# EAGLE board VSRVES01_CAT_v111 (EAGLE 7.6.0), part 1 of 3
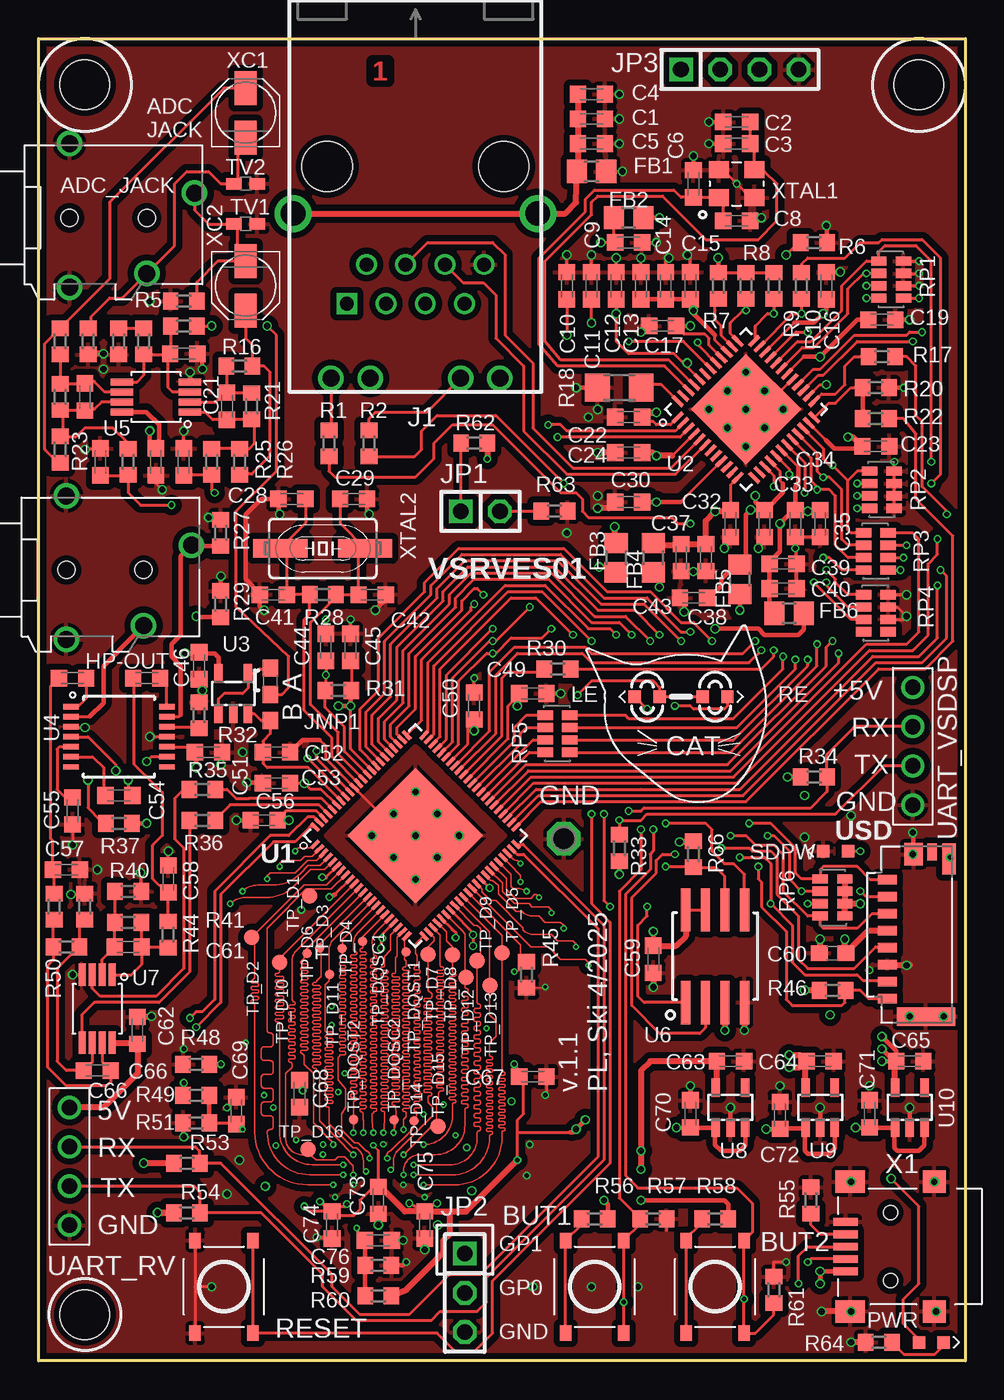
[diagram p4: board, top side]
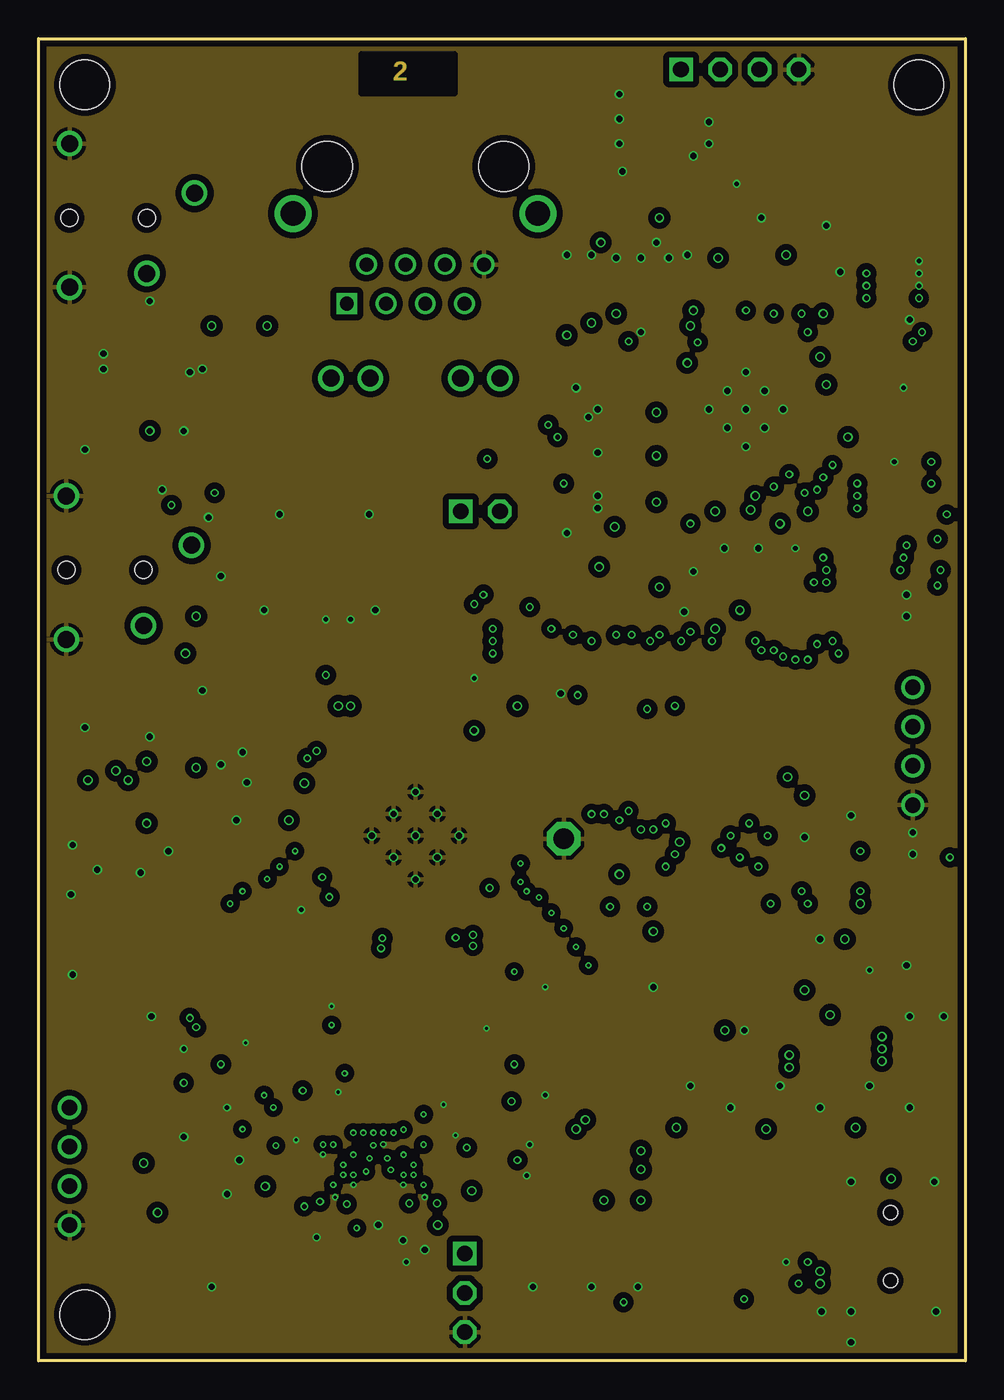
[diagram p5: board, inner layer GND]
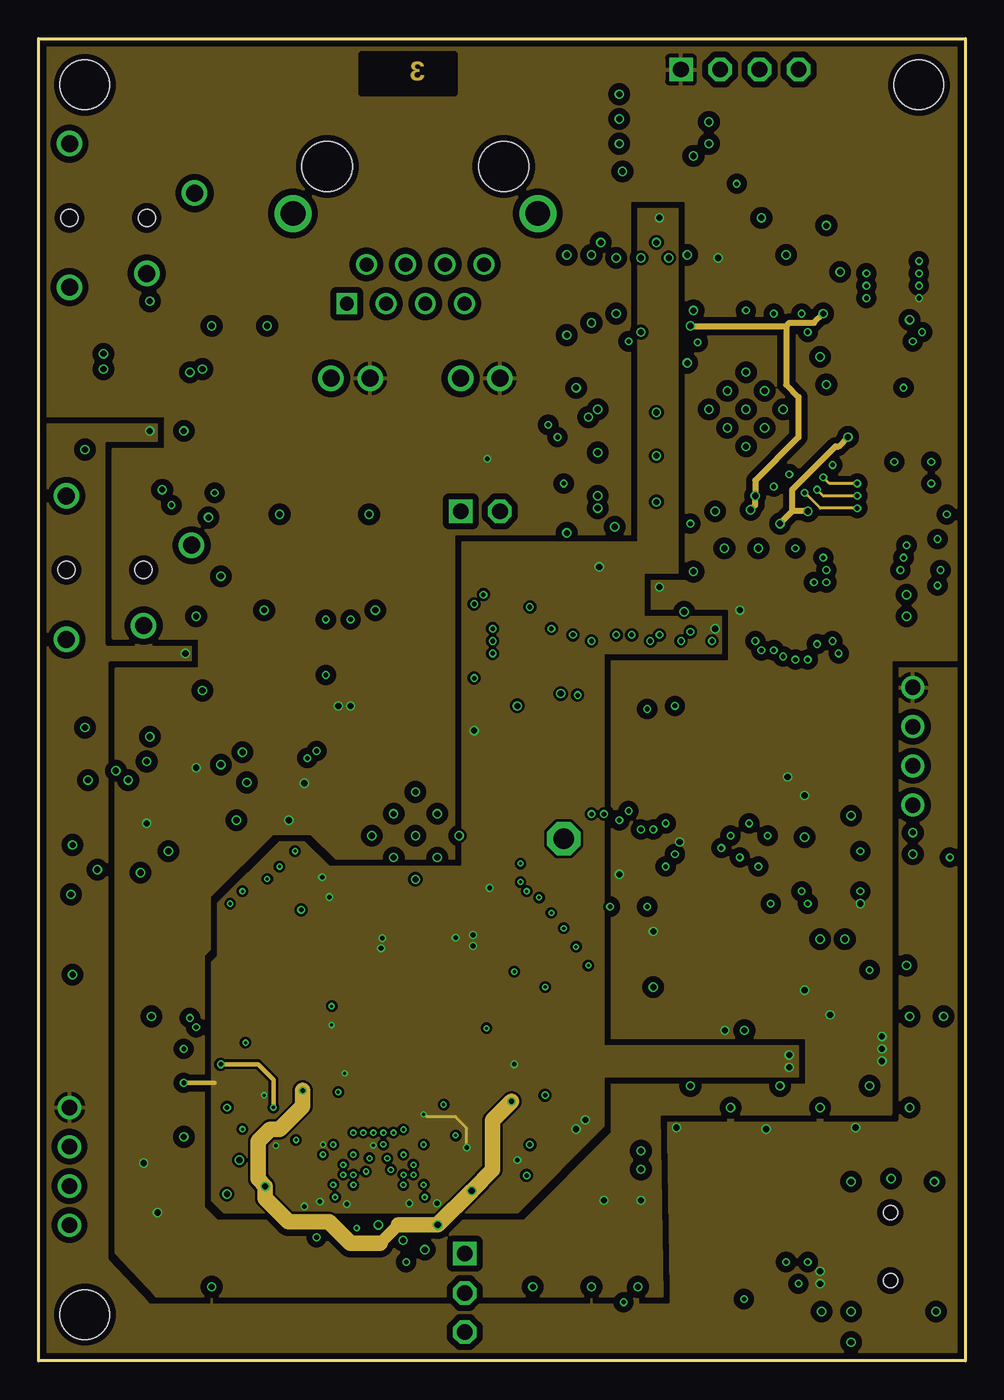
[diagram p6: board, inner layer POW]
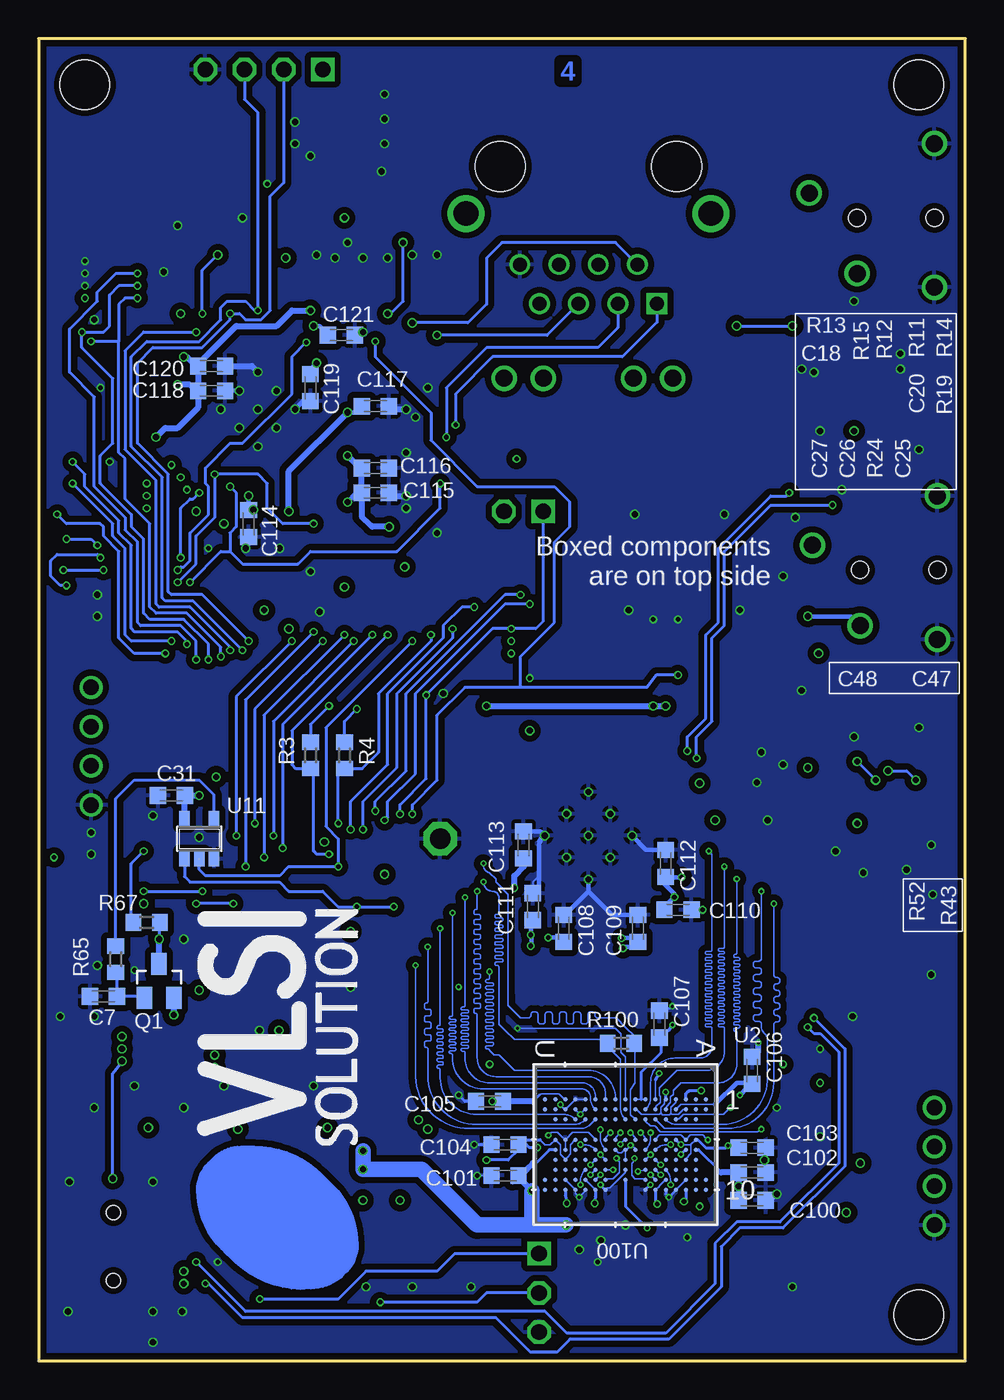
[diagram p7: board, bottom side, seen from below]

Size 60 x 85.6 mm. Coordinates in mm from the lower left corner, seen from the top.
Outline: 0,0 0,85.6 60,85.6 60,0 0,0
Copper layers (1*2+15*16): Top 0.035mm / dielectric 0.12mm / GND 0.0175mm / dielectric 1.2mm / POW 0.0175mm / dielectric 0.12mm / Bottom 0.035mm
Design rules "4L_JLC_tight_Eagle_Rule *": minimum track width 0.1mm, minimum drill 0.2mm, track to track 0.1mm, track to pad 0.1mm, pad to pad 0.15mm, via to via 0.2mm, smd to smd 0mil, copper to edge 6mil, drill to drill 12mil, minimum pad ring 0.1mm, minimum via ring 4mil, stop-mask expansion 2mil, vias tented up to drill 25mil, thermal gap 10mil
Holes 3.2 mm at 57,82.6 3,3 3,82.6
Milling: 4 lines

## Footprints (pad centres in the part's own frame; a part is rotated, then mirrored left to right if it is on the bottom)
SJ-43514B = drill 1.1: 1 8.1,1.6; 4 5,-3.6; 5 0,4.8; 6 0,-4.5 | hole 1.1: 0,0; 5,0
SW_SMD-SW-4_5.1X5.1X2.5_TS-1187A-C-E-B = smd 1 x 0.75: P1 -3,1.875; P2 3,1.875; S1 -3,-1.875; S2 3,-1.875
C0603K = smd 1.05 x 1.08: 1 -0.875,0; 2 0.875,0
C0603 = smd 1.1 x 1: 1 -0.85,0; 2 0.85,0
L0805 = smd 1.3 x 1.5: 1 -0.95,0; 2 0.95,0
JXD7 = drill 1.1: L1 -5.465,13.72; L2 -2.925,13.72; L3 2.925,13.72; L4 5.465,13.72 | drill 0.9 square: P1 4.445,8.89 | drill 0.9: P2 3.175,6.35; P3 1.905,8.89; P4 0.635,6.35; P5 -0.635,8.89; P6 -1.905,6.35; P7 -3.175,8.89; P8 -4.445,6.35 | drill 1.6: S1 7.925,3.05; S2 -7.925,3.05 | hole 3.25: 5.715,0; -5.715,0
0603X2 = smd 1.1 x 1: 1 -0.85,0; 2 0.85,0; 3 2.55,0
1X02 = drill 1.016 square: 1 -1.27,0 | drill 1.016 octagon: 2 1.27,0
1X03 = drill 1.016 square: 1 -2.54,0 | drill 1.016 octagon: 2 0,0; 3 2.54,0
1X04 = drill 1.016 square: 1 -3.81,0 | drill 1.016 octagon: 2 -1.27,0; 3 1.27,0; 4 3.81,0
LED_0603 = smd 0.8 x 0.8: A 0.8,0; C -0.8,0
SOT23 = smd 1.4 x 1: 1 1.1,-0.95; 2 1.1,0.95; 3 -1.1,0
R0603 = smd 1 x 1.1: 1 -0.85,0; 2 0.85,0
R1206 = smd 1.6 x 1.803: 1 -1.422,0; 2 1.422,0
RAS_ARR_1206 = smd 1 x 0.6: 1 -0.8,1.2; 2 0.8,1.2; 3 -0.8,0.4; 4 0.8,0.4; 5 -0.8,-0.4; 6 0.8,-0.4; 7 -0.8,-1.2; 8 0.8,-1.2
P1-13 = drill 1.321 pad 2.159 octagon: TP 0,0
TP10R = smd 1 x 1: TP 0,0
TP06R = smd 0.6 x 0.6: TP 0,0
0603 = smd 1.02 x 0.76: 1 -0.76,0; 2 0.76,0
QFN88_NEW2Q = smd 0.23 x 0.7: 1 -4.2,-5; 2 -3.8,-5; 3 -3.4,-5; 4 -3,-5; 5 -2.6,-5; 6 -2.2,-5; 7 -1.8,-5; 8 -1.4,-5; 9 -1,-5; 10 -0.6,-5; 11 -0.2,-5; 12 0.2,-5; 13 0.6,-5; 14 1,-5; 15 1.4,-5; 16 1.8,-5; 17 2.2,-5; 18 2.6,-5; 19 3,-5; 20 3.4,-5; 21 3.8,-5; 22 4.2,-5; 45 4.2,5; 46 3.8,5; 47 3.4,5; 48 3,5; 49 2.6,5; 50 2.2,5; 51 1.8,5; 52 1.4,5; 53 1,5; 54 0.6,5; 55 0.2,5; 56 -0.2,5; 57 -0.6,5; 58 -1,5; 59 -1.4,5; 60 -1.8,5; 61 -2.2,5; 62 -2.6,5; 63 -3,5; 64 -3.4,5; 65 -3.8,5; 66 -4.2,5 | smd 0.7 x 0.23: 23 5,-4.2; 24 5,-3.8; 25 5,-3.4; 26 5,-3; 27 5,-2.6; 28 5,-2.2; 29 5,-1.8; 30 5,-1.4; 31 5,-1; 32 5,-0.6; 33 5,-0.2; 34 5,0.2; 35 5,0.6; 36 5,1; 37 5,1.4; 38 5,1.8; 39 5,2.2; 40 5,2.6; 41 5,3; 42 5,3.4; 43 5,3.8; 44 5,4.2; 67 -5,4.2; 68 -5,3.8; 69 -5,3.4; 70 -5,3; 71 -5,2.6; 72 -5,2.2; 73 -5,1.8; 74 -5,1.4; 75 -5,1; 76 -5,0.6; 77 -5,0.2; 78 -5,-0.2; 79 -5,-0.6; 80 -5,-1; 81 -5,-1.4; 82 -5,-1.8; 83 -5,-2.2; 84 -5,-2.6; 85 -5,-3; 86 -5,-3.4; 87 -5,-3.8; 88 -5,-4.2 | smd 6.2 x 6.2: GNDPAD 0,0 | drill 0.4: P$1 -2,2; P$2 0,2; P$3 2,2; P$4 -2,0; P$5 0,0; P$6 2,0; P$7 -2,-2; P$8 0,-2; P$9 2,-2
48-VFQFN_7X7 = smd 0.9 x 0.25: 1 -3.5,2.75; 2 -3.5,2.25; 3 -3.5,1.75; 4 -3.5,1.25; 5 -3.5,0.75; 6 -3.5,0.25; 7 -3.5,-0.25; 8 -3.5,-0.75; 9 -3.5,-1.25; 10 -3.5,-1.75; 11 -3.5,-2.25; 12 -3.5,-2.75; 25 3.5,-2.75; 26 3.5,-2.25; 27 3.5,-1.75; 28 3.5,-1.25; 29 3.5,-0.75; 30 3.5,-0.25; 31 3.5,0.25; 32 3.5,0.75; 33 3.5,1.25; 34 3.5,1.75; 35 3.5,2.25; 36 3.5,2.75 | smd 0.25 x 0.9: 13 -2.75,-3.5; 14 -2.25,-3.5; 15 -1.75,-3.5; 16 -1.25,-3.5; 17 -0.75,-3.5; 18 -0.25,-3.5; 19 0.25,-3.5; 20 0.75,-3.5; 21 1.25,-3.5; 22 1.75,-3.5; 23 2.25,-3.5; 24 2.75,-3.5; 37 2.75,3.5; 38 2.25,3.5; 39 1.75,3.5; 40 1.25,3.5; 41 0.75,3.5; 42 0.25,3.5; 43 -0.25,3.5; 44 -0.75,3.5; 45 -1.25,3.5; 46 -1.75,3.5; 47 -2.25,3.5; 48 -2.75,3.5 | smd 5.05 x 5.05: 49 0,0 | drill 0.4: G1 -1.7,1.7; G2 0,1.7; G3 1.7,1.7; G4 -1.7,0; G5 0,0; G6 1.7,0; G7 -1.7,-1.7; G8 0,-1.7; G9 1.7,-1.7
SOT23-5 = smd 0.55 x 1.2: 1 -0.95,-1.3; 2 0,-1.3; 3 0.95,-1.3; 4 0.95,1.3; 5 -0.95,1.3
TSSOP-14_4.4MM = smd 0.35 x 1: 1 -1.95,-3.1; 2 -1.3,-3.1; 3 -0.65,-3.1; 4 0,-3.1; 5 0.65,-3.1; 6 1.3,-3.1; 7 1.95,-3.1; 8 1.95,3.1; 9 1.3,3.1; 10 0.65,3.1; 11 0,3.1; 12 -0.65,3.1; 13 -1.3,3.1; 14 -1.95,3.1
8-VSSOP = smd 0.45 x 1.45: 1 -0.975,-2.2; 2 -0.325,-2.2; 3 0.325,-2.2; 4 0.975,-2.2; 5 0.975,2.2; 6 0.325,2.2; 7 -0.325,2.2; 8 -0.975,2.2
SO-08M_WIDE = smd 0.6 x 2.8: 1 -1.905,-3; 2 -0.635,-3; 3 0.635,-3; 4 1.905,-3; 5 1.905,3; 6 0.635,3; 7 -0.635,3; 8 -1.905,3
SOT23-5L = smd 0.55 x 1.2: 1 -0.95,-1.3; 2 0,-1.3; 3 0.95,-1.3; 4 0.95,1.3; 5 -0.95,1.3
SOT23-5' = smd 0.69 x 0.99: 1 -0.95,-1.29; 2 0,-1.29; 3 0.95,-1.29; 4 0.95,1.3; 5 -0.95,1.3
FBGA134_ISI-L = smd 0.305 x 0.305: A1 -2.925,5.2; A2 -2.275,5.2; A9 2.275,5.2; A10 2.925,5.2; B1 -2.925,4.55; B2 -2.275,4.55; B3 -1.625,4.55; B5 -0.325,4.55; B6 0.325,4.55; B7 0.975,4.55; B8 1.625,4.55; B9 2.275,4.55; B10 2.925,4.55; C1 -2.925,3.9; C2 -2.275,3.9; C3 -1.625,3.9; C5 -0.325,3.9; C6 0.325,3.9; C7 0.975,3.9; C8 1.625,3.9; C9 2.275,3.9; C10 2.925,3.9; D1 -2.925,3.25; D2 -2.275,3.25; D3 -1.625,3.25; D5 -0.325,3.25; D6 0.325,3.25; D7 0.975,3.25; D8 1.625,3.25; D9 2.275,3.25; D10 2.925,3.25; E1 -2.925,2.6; E2 -2.275,2.6; E3 -1.625,2.6; E5 -0.325,2.6; E6 0.325,2.6; E7 0.975,2.6; E8 1.625,2.6; E9 2.275,2.6; E10 2.925,2.6; F1 -2.925,1.95; F2 -2.275,1.95; F3 -1.625,1.95; F5 -0.325,1.95; F6 0.325,1.95; F7 0.975,1.95; F8 1.625,1.95; F9 2.275,1.95; F10 2.925,1.95; G1 -2.925,1.3; G2 -2.275,1.3; G3 -1.625,1.3; G5 -0.325,1.3; G6 0.325,1.3; G7 0.975,1.3; G8 1.625,1.3; G9 2.275,1.3; G10 2.925,1.3; H1 -2.925,0.65; H2 -2.275,0.65; H3 -1.625,0.65; H5 -0.325,0.65; H6 0.325,0.65; J1 -2.925,0; J2 -2.275,0; J3 -1.625,0; J5 -0.325,0; J6 0.325,0; J7 0.975,0; J8 1.625,0; J9 2.275,0; K1 -2.925,-0.65; K2 -2.275,-0.65; K3 -1.625,-0.65; K5 -0.325,-0.65; K6 0.325,-0.65; L1 -2.925,-1.3; L2 -2.275,-1.3; L3 -1.625,-1.3; L5 -0.325,-1.3; L6 0.325,-1.3; L7 0.975,-1.3; L8 1.625,-1.3; L9 2.275,-1.3; L10 2.925,-1.3; M1 -2.925,-1.95; M2 -2.275,-1.95; M3 -1.625,-1.95; M5 -0.325,-1.95; M6 0.325,-1.95; M7 0.975,-1.95; M8 1.625,-1.95; M9 2.275,-1.95; M10 2.925,-1.95; N1 -2.925,-2.6; N2 -2.275,-2.6; N3 -1.625,-2.6; N5 -0.325,-2.6; N6 0.325,-2.6; N7 0.975,-2.6; N8 1.625,-2.6; N9 2.275,-2.6; N10 2.925,-2.6; P1 -2.925,-3.25; P2 -2.275,-3.25; P3 -1.625,-3.25; P5 -0.325,-3.25; P6 0.325,-3.25; P7 0.975,-3.25; P8 1.625,-3.25; P9 2.275,-3.25; P10 2.925,-3.25; R1 -2.925,-3.9; R2 -2.275,-3.9; R3 -1.625,-3.9; R5 -0.325,-3.9; R6 0.325,-3.9; R7 0.975,-3.9; R8 1.625,-3.9; R9 2.275,-3.9; R10 2.925,-3.9; T1 -2.925,-4.55; T2 -2.275,-4.55; T3 -1.625,-4.55; T5 -0.325,-4.55; T6 0.325,-4.55; T7 0.975,-4.55; T8 1.625,-4.55; T9 2.275,-4.55; T10 2.925,-4.55; U1 -2.925,-5.2; U2 -2.275,-5.2; U9 2.275,-5.2; U10 2.925,-5.2
4X1_2.54MM_CON = drill 1: P$1 0,0; P$2 2.54,0; P$3 5.08,0; P$4 7.62,0
47(309/571) = smd 0.6 x 1.25: 1 -3.55,-1.45; 2 -2.45,-1.45; 3 -1.35,-1.45; 4 -0.25,-1.45; 5 0.85,-1.45; 6 1.95,-1.45; 7 3.05,-1.45; 8 4.15,-1.45 | smd 1.2 x 3.79: 9 5.3,1.05 | smd 1.45 x 1.2: 10 -5.2,0.25 | smd 1.1 x 0.6: 11 -5.35,1.45 | smd 2 x 0.85: 12 -4.9,2.55
MINI_USB_KOREAN_HROPARTS_U-M-M5SS-W-2_C91144 = smd 1.6 x 0.5: 1 -4.15,-1.6; 2 -4.15,-0.8; 3 -4.15,0; 4 -4.15,0.8; 5 -4.15,1.6 | smd 1.9 x 1.45: G1 -3.85,-4.2; G2 -3.85,4.2 | smd 1.5 x 1.45: G3 1.6,-4.2; G4 1.6,4.2 | hole 0.9: -1.25,2.2; -1.25,-2.2
EC-SMD-44X44 = smd 2.2 x 1.4: + 1.6,0; - -1.6,0
3.2X2.5_CRYSTAL = smd 1.3 x 1.1: 1 -1.15,-0.9; 2 1.15,-0.9; 3 1.15,0.9; 4 -1.15,0.9
CSM-3X = smd 3.5 x 1.2: 1 -2.75,0; 2 2.75,0

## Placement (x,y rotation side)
$$U$1  [KISSA]  39.2,39.8 0 top
ADC_JACK  CON_3M5_4WAY_JACK-TH  [SJ-43514B]  2,74 0 top
BUT1  SW_SMD-C318887  [SW_SMD-SW-4_5.1X5.1X2.5_TS-1187A-C-E-B]  36,4.8 90 top
BUT2  SW_SMD-C318887  [SW_SMD-SW-4_5.1X5.1X2.5_TS-1187A-C-E-B]  43.8,4.8 90 top
C1  100nF  [C0603K]  35.8,80.4 0 top
C2  12p  [C0603K]  45.2,80.2 180 top
C3  12p  [C0603K]  45.2,78.8 180 top
C4  100nF  [C0603K]  35.8,82 0 top
C5  100nF  [C0603K]  35.8,78.8 0 top
C6  12p  [C0603K]  42.4,76.2 90 top
C7  100nF  [C0603K]  55.8,23.6 180 bottom
C8  12p  [C0603K]  45.2,73.8 0 top
C9  10u/6.3v  [C0603K]  38.2,72.4 0 top
C10  100nF  [C0603K]  34.2,69.6 90 top
C11  100nF  [C0603K]  35.8,69.6 90 top
C12  100nF  [C0603K]  37.4,69.6 90 top
C13  10u/6.3v  [C0603K]  39,69.6 90 top
C14  100nF  [C0603K]  40.6,69.6 90 top
C15  10nF  [C0603K]  42.2,69.6 90 top
C16  10nF  [C0603K]  51,69.6 90 top
C17  10nF  [C0603K]  40.4,67 180 top
C18  1uF  [C0603K]  9.4,65.2 0 top
C19  10nF  [C0603K]  54.6,67.4 0 top
C20  100pF  [C0603K]  3,62.4 270 top
C21  100pF  [C0603K]  12.2,61.8 270 top
C22  10nF  [C0603K]  38.2,61.1 180 top
C23  10nF  [C0603K]  54.2,59.2 0 top
C24  10nF  [C0603K]  38.2,58.8 180 top
C25  1n/NP0  [C0603K]  4,58.2 90 top
C26  100nF  [C0603K]  7.6,58.2 270 top
C27  1n/NP0  [C0603K]  9.4,58.2 90 top
C28  12p  [C0603K]  16.4,55.8 0 top
C29  12p  [C0603K]  20.4,55.8 180 top
C30  10nF  [C0603K]  38.2,55.6 180 top
C31  100nF  [C0603K]  51.4,36.6 180 bottom
C32  10nF  [C0603K]  44.8,54.2 270 top
C33  10nF  [C0603K]  47,54.2 270 top
C34  10nF  [C0603K]  49,54.2 270 top
C35  100nF  [C0603K]  50.6,54.2 270 top
C37  10u/6.3v  [C0603K]  41.6,52 270 top
C38  100nF  [C0603K]  43.2,52 270 top
C39  10u/6.3v  [C0603K]  48.2,51.6 0 top
C40  10u/6.3v  [C0603K]  48.2,50 0 top
C41  12p  [C0603K]  15.2,49.6 0 top
C42  12p  [C0603K]  21.6,49.6 180 top
C43  10u/6.3v  [C0603K]  42.4,49.4 180 top
C44  100nF  [C0603K]  18.6,46.2 90 top
C45  100nF  [C0603K]  20.2,46.2 90 top
C46  100nF  [C0603K]  10.4,45 270 top
C47  2.2uF  [C0603K]  2.2,44.2 0 top
C48  2.2uF  [C0603K]  7,44.2 0 top
C49  4.7uF  [C0603K]  32,43.2 0 top
C50  100nF  [C0603K]  28.2,42.4 90 top
C51  1uF  [C0603K]  11,39.4 0 top
C52  1uF  [C0603K]  15.4,39.4 0 top
C53  100nF  [C0603K]  15.4,37.4 180 top
C54  1uF  [C0603K]  5.2,36.6 180 top
C55  1uF  [C0603K]  2.2,35.6 270 top
C56  4.7uF  [C0603K]  14.6,35 180 top
C57  3.3n/NP0  [C0603K]  1.8,31.8 0 top
C58  3.3n/NP0  [C0603K]  8.4,31.2 90 top
C59  100nF  [C0603K]  39.8,26 270 top
C60  1uF  [C0603]  51.4,26.4 180 top
C61  1n/NP0  [C0603K]  5.8,26.8 0 top
C62  100nF  [C0603K]  6.4,21.4 90 top
C63  1uF  [C0603K]  44.8,19.4 0 top
C64  1uF  [C0603K]  50.6,19.4 0 top
C65  1uF  [C0603K]  56.4,19.4 0 top
C66  1n/NP0  [C0603K]  3.8,18.8 0 top
C67  100nF  [C0603K]  32,18.4 0 top
C68  100nF  [C0603K]  16.9,17.3 270 top
C69  100nF  [C0603K]  12.8,16.2 90 top
C70  1uF  [C0603K]  42.2,16 90 top
C71  1uF  [C0603K]  53.8,16 90 top
C72  1uF  [C0603K]  48,15.9 90 top
C73  100nF  [C0603K]  22,10.4 270 top
C74  100nF  [C0603K]  19,8.8 270 top
C75  10u/6.3v  [C0603K]  25,8.8 270 top
C76  100nF  [C0603K]  22,7.8 0 top
C100  10u/6.3v  [C0603K]  13.8,10.4 0 bottom
C101  100nF  [C0603K]  29.8,12 180 bottom
C102  100nF  [C0603K]  13.8,12.2 0 bottom
C103  100nF  [C0603K]  13.8,13.8 0 bottom
C104  100nF  [C0603K]  29.8,14 180 bottom
C105  100nF  [C0603K]  30.8,16.8 180 bottom
C106  100nF  [C0603K]  13.8,18.8 90 bottom
C107  100nF  [C0603K]  19.8,21.8 90 bottom
C108  100nF  [C0603K]  26,28 90 bottom
C109  100nF  [C0603K]  21.2,28 90 bottom
C110  4.7uF  [C0603K]  18.6,29.2 0 bottom
C111  100nF  [C0603K]  28,29.4 90 bottom
C112  4.7uF  [C0603K]  19.4,32.2 90 bottom
C113  100nF  [C0603K]  28.6,33.4 90 bottom
C114  100nF  [C0603K]  46.4,54.2 270 bottom
C115  100nF  [C0603K]  38.2,56.2 0 bottom
C116  10u/6.3v  [C0603K]  38.2,57.8 0 bottom
C117  10u/6.3v  [C0603K]  38.2,61.8 0 bottom
C118  10u/6.3v  [C0603K]  48.8,62.8 0 bottom
C119  10nF  [C0603K]  42.4,63 270 bottom
C120  10nF  [C0603K]  48.8,64.4 0 bottom
C121  10u/6.3v  [C0603K]  40.4,66.4 0 bottom
FB1  BLM21P221SG  [L0805]  35.8,77 0 top
FB2  BLM21P221SG  [L0805]  38.2,74 180 top
FB3  BLM21P221SG  [L0805]  37.4,52 90 top
FB4  BLM21P221SG  [L0805]  39.8,52 90 top
FB5  BLM21P221SG  [L0805]  45.4,50.6 90 top
FB6  BLM21P221SG  [L0805]  48.6,48.4 180 top
HP-OUT  CON_3M5_4WAY_JACK-TH  [SJ-43514B]  1.8,51.2 0 top
J1  JXD7-0V0XNL08NL  [JXD7]  24.4,77.33 180 top
JMP1  0R-JMPR  [0603X2]  15,44 270 top
JP1  dnc  [1X02]  28.6,55 0 top
JP2  3PIN  [1X03]  27.6,4.4 270 top
JP3  dnc  [1X04]  45.4,83.6 0 top
LE  amber  [LED_0603]  39.4,43 0 top
PWR  green  [LED_0603]  57.8,1.2 180 top
Q1  CJ3401A  [SOT23]  52.2,24.6 270 bottom
R1  1k  [R0603]  18.8,59.4 270 top
R2  1k  [R0603]  21.4,59.4 270 top
R3  1k  [R0603]  42.4,39.2 90 bottom
R4  1k  [R0603]  40.2,39.2 90 bottom
R5  100k  [R0603]  9.4,68.6 0 top
R6  1k  [R0603]  50.2,72.4 180 top
R7  10k  [R0603]  44,69.6 90 top
R8  10k  [R0603]  45.8,69.6 90 top
R9  10k  [R0603]  47.6,69.6 90 top
R10  10  [R0603]  49.4,69.6 90 top
R11  100k  [R0603]  3.2,66 90 top
R12  470k  [R0603]  5.2,66 90 top
R13  8k2  [R0603]  9.4,67 180 top
R14  8.2k  [R0603]  1.4,66 270 top
R15  470k  [R0603]  6.8,66 270 top
R16  8.2k  [R0603]  13,64.4 180 top
R17  10  [R0603]  54.6,65 0 top
R18  6.04k  [R1206]  37.6,63 180 top
R19  8.2k  [R0603]  1.4,62.4 270 top
R20  dnc  [R0603]  54.2,63 180 top
R21  8.2k  [R0603]  13.8,61.8 270 top
R22  10  [R0603]  54.2,61 0 top
R23  dnc  [R0603]  1.4,59 90 top
R24  100  [R0603]  5.8,58.2 270 top
R25  100  [R0603]  11.2,58.2 270 top
R26  dnc  [R0603]  13,58.2 90 top
R27  100k  [R0603]  11.8,53.6 270 top
R28  470k  [R0603]  18.4,49.6 0 top
R29  100k  [R0603]  11.8,49 270 top
R30  10  [R0603]  33.6,44.8 180 top
R31  100k  [R0603]  19.4,43.4 0 top
R32  82k  [R0603]  10.4,41.8 90 top
R33  10k  [R0603]  37.6,33.2 270 top
R34  10k  [R0603]  50.2,37.8 180 top
R35  1k  [R0603]  10.6,37 180 top
R36  1k  [R0603]  10.6,35 180 top
R37  10k  [R0603]  5.2,34.8 0 top
R40  470k  [R0603]  5.8,30.4 180 top
R41  1k  [R0603]  5.8,28.4 0 top
R43  1k  [R0603]  1,29.4 90 top
R44  1k  [R0603]  8.4,27.6 90 top
R45  10k  [R0603]  31.6,25 90 top
R46  10k  [R0603]  51.4,24 180 top
R48  240  [R0603]  10.2,19.2 0 top
R49  2k  [R0603]  10.2,17.2 180 top
R50  1k  [R0603]  1.8,26.8 180 top
R51  2k  [R0603]  10.2,15.4 0 top
R52  470k  [R0603]  3,29.4 270 top
R53  10k  [R0603]  9.6,12.8 180 top
R54  10k  [R0603]  9.6,9.6 180 top
R55  100k  [R0603]  50,10.4 90 top
R56  10k  [R0603]  36,9.2 0 top
R57  100k  [R0603]  39.8,9.2 180 top
R58  10k  [R0603]  43.8,9.2 0 top
R59  2k  [R0603]  22,6.2 180 top
R60  2k  [R0603]  22,4.2 0 top
R61  100k  [R0603]  47.6,4.6 270 top
R62  100k  [R0603]  28.2,59.4 0 top
R63  10k  [R0603]  33.4,55 180 top
R64  2k  [R0603]  54.4,1.2 0 top
R65  1k  [R0603]  55,26 270 bottom
R66  100k  [R0603]  42.4,32.8 90 top
R67  2k  [R0603]  53,28.4 180 bottom
R100  100  [R0603]  22.29,20.55 0 bottom
RE  green  [LED_0603]  43.8,43 180 top
RESET  SW_SMD-C318887  [SW_SMD-SW-4_5.1X5.1X2.5_TS-1187A-C-E-B]  12,4.8 90 top
RP1  10k  [RAS_ARR_1206]  55.2,70 180 top
RP2  1k  [RAS_ARR_1206]  54.6,56.4 180 top
RP3  10  [RAS_ARR_1206]  54.2,52.4 180 top
RP4  1k  [RAS_ARR_1206]  54.2,48.4 180 top
RP5  10  [RAS_ARR_1206]  33.6,40.6 180 top
RP6  10k  [RAS_ARR_1206]  51.4,30 0 top
SDPW  green  [LED_0603]  51.6,33 0 top
TP1  TPPAD1-13  [P1-13]  34,33.8 180 top
TP_D1  TPTP10R  [TP10R]  17.53,30.09 0 top
TP_D2  TPTP10R  [TP10R]  13.8,27.4 0 top
TP_D3  TPTP06R  [TP06R]  18.18,26.75 0 top
TP_D4  TPTP06R  [TP06R]  19.64,26.71 0 top
TP_D5  TPTP10R  [TP10R]  30,26.4 0 top
TP_D6  TPTP06R  [TP06R]  17.38,26.37 0 top
TP_D7  TPTP10R  [TP10R]  25.2,26.3 0 top
TP_D8  TPTP10R  [TP10R]  26.8,26.28 0 top
TP_D9  TPTP10R  [TP10R]  28.39,25.91 0 top
TP_D10  TPTP10R  [TP10R]  15.6,25.79 0 top
TP_D11  TPTP06R  [TP06R]  18.83,25.01 0 top
TP_D12  TPTP10R  [TP10R]  27.67,24.81 0 top
TP_D13  TPTP10R  [TP10R]  29.24,24.3 0 top
TP_D14  TPTP06R  [TP06R]  24.31,15.55 0 top
TP_D15  TPTP10R  [TP10R]  25.85,15.19 0 top
TP_D16  TPTP10R  [TP10R]  17.45,13.71 0 top
TP_DQSC1  TPTP06R  [TP06R]  20.99,27.16 0 top
TP_DQSC2  TPTP06R  [TP06R]  23,15.6 0 top
TP_DQST1  TPTP06R  [TP06R]  23.8,26.46 0 top
TP_DQST2  TPTP06R  [TP06R]  20.39,15.62 0 top
TV1  CG0603MLA-5.5ME  [0603]  13.4,73.6 0 top
TV2  CG0603MLA-5.5ME  [0603]  13.4,76.2 0 top
U1  VSRVES01  [QFN88_NEW2Q]  24.4,34 315 top
U2  KSZ9131RNX  [48-VFQFN_7X7]  45.8,61.6 45 top
U3  TLV172-DBV  [SOT23-5]  12.6,43.2 0 top
U4  TPA6139A2  [TSSOP-14_4.4MM]  5.2,40.4 270 top
U5  TLV2172IDGKR_8VSSOP  [8-VSSOP]  7.6,62.4 90 top
U6  SPI_FLASH_WIDE_AND_NARROW  [SO-08M_WIDE]  43.8,26.2 0 top
U7  TLV2172IDGKR_8VSSOP  [8-VSSOP]  3.8,22.8 180 top
U8  LP5907MFX-1.8  [SOT23-5L]  44.8,16.4 0 top
U9  TLV70212DBVR  [SOT23-5L]  50.6,16.4 0 top
U10  ME6211C33M5G  [SOT23-5L]  56.4,16.4 0 top
U11  74AHC1G08DBV  [SOT23-5']  49.6,33.8 0 bottom
U100  IS43LD16640C-25BLIFBGA134_ISI-L  [FBGA134_ISI-L]  22,14 270 bottom
U$100  [LOGO]  39,4.4 90 bottom
UART_RV  4X1_2.54MM_CON  [4X1_2.54MM_CON]  2,16.4 270 top
UART_VSDSP  4X1_2.54MM_CON  [4X1_2.54MM_CON]  56.6,43.6 270 top
USD  CON-USD-AB  [47(309/571)]  56.4,27.6 270 top
X1  USB_MINI_KOREAN_U-M-M5SS-W-2_C91144  [MINI_USB_KOREAN_HROPARTS_U-M-M5SS-W-2_C91144]  56.4,7.4 0 top
XC1  10uF/16V  [EC-SMD-44X44]  13.4,80.8 90 top
XC2  10uF/16V  [EC-SMD-44X44]  13.4,69.6 270 top
XTAL1  3.2X2.5_C9006_25MHz  [3.2X2.5_CRYSTAL]  45.2,76.2 0 top
XTAL2  12.288MHz/20p  [CSM-3X]  18.4,52.6 0 top

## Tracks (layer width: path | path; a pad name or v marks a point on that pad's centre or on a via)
1.2V  (via drill 0.2, 0.3, 0.4)
  Top 0.11: 18.86,9.68 C74.1 19.07,9.68 19.2,9.8 19.4,10 | 24.93,9.68 C75.1 25,9.8 | 22,13.6 v21.67,13.96 | 22.4,11 22.27,11 C73.1 21.68,11.28 | 31.4,18.12 C67.1 31.12,18.68 | 28.2,27.65 v28.13,27.58 | 19.2,30.21 19.2,30.2
  Top 0.2: 18.86,9.68 v18.22,10.31 | 19.4,10 19.8,10 v19.95,10.15 | 24.93,9.68 v24,10.2 | 25,9.8 v25.8,10.2 | C73.1 22,13.6 | 21.68,11.28 20.8,10.4 20.8,9.8 20.4,9.4 19.6,9.4 19.2,9.8 | v31,13 31,14.8 | 31,14.8 31,15.6 31.4,16 31.4,18.12 | 31.12,18.68 v30.8,19.2 | R49.2 9.36,17 | C74.1 17.52,9.68 v17.2,10 | 31,14.8 34.4,14.8 | U1.29 28.2,27.65 | v28.13,27.58 v28.13,26.86 | U1.60 27.8,39.95 27.8,40.92 | 27.8,40.92 27.8,41.4 | v28.2,40.8 C50.1 27.8,40.92 | U1.6 18.59,31.3 | U1.9 19.2,30.21 | U1.27 26.72,28 26.81,27.91 27.01,27.71 v27,27.4 | U1.36 v29.2,30.61 | FB3.1 37.4,51.2 | U1.19 22.25,27.61 v22.25,27.37 | v22.17,26.71 22.2,26.74 22.2,27.4
  Top 0.3: v35.4,15.6 v34.8,15 34.6,14.8 34.4,14.8 | 18.59,31.3 v18.36,31.31 | 19.2,30.2 v18.83,30.03 | FB6.1 49.55,47.35 49.2,47 47,47 46.6,47.4 v43.8,47.4 | FB2.1 v40.2,74 | C64.1 49.65,19.32 49.65,19.55 | R49.2 9.4,17.25 v9.4,18
  Top 0.4: 24.93,9.68 23.73,9.68 22.4,11 | C75.1 26.6,9.68 | 26.6,9.68 27.68,9.68 v31,13 | R60.2 23.8,4.6 26.2,7 26.2,7.8 26.6,8.2 26.6,9.68 | 37.4,51.2 37.4,51.4 v36.3,51.4 | U9.5 49.65,19.32 | v48.6,19 49.23,19 C64.1 | v48.6,19.8 49.3,19.8 49.8,19.4
  POW 0.2: v27.72,13.81 27.72,15.07 27,15.8 25.18,15.8 v24.93,15.96
  POW 0.3: v9.4,18 11.4,18
  Bottom 0.11: U100.H1 20.97,16.93 U100.G1 | 19.69,19.98 19.69,20.04 | U100.F1 20.05,18.17 | 19.69,20.84 C107.1 | U100.D2 18.73,16.27 18.4,16.6 16.2,16.6 | C106.1 13.88,17.93 | U100.C7 18.1,13.08 17.76,13.42 17.76,14.02 | 17.76,14.02 U100.B5 | 15.12,14.32 15,14.2 15,14.12 C103.1 15.21,13.8 | 20.05,10.25 v19.95,10.15 | U100.E9 19.41,11.72 19.82,11.32 19.82,11.3 U100.F10 | U100.P2 25.27,16.27 v24.93,15.96 24.61,16.27 U100.N2 | 25.25,14.38 U100.P5 25.27,14.32 25.58,14 25.58,13.4 25.73,13.2 U100.R7 25.9,13.05 26.22,13.37 26.22,13.99 U100.T5 26.88,14 27.2,14 27.52,14.32 | C104.1 28.6,14.32 28.12,14.32 | U100.N9 24.25,11.36 24.23,11.36 U100.M10 | 27.69,13.8 v27.72,13.81 | U100.H6 21.35,13.75 v21.67,13.96 21.93,13.68 U100.J6 | U100.J7 U100.J6 | U100.D5 18.73,14.32 | v18.42,14 17.77,14 17.76,14.02 | C104.1 28.93,13.68 | 15.5,13.8 v15.36,13.94 | U100.J6 22.05,13.68 22.26,13.47 22.45,13.47 U100.K6 | 28.4,14 C104.1 | C112.1 18.98,31.3 | C110.1 19.48,29.39 | 28.73,32.4 C113.1 28.6,32
  Bottom 0.2: 20.97,16.93 20.97,18.7 19.69,19.98 | 20.05,18.17 v19.82,18.62 | 19.69,20.04 19.69,20.84 | U100.F10 20.05,10.25 | U100.C10 18.1,10.43 v18.22,10.31 | 15.21,13.8 v15.36,13.94 | U100.M10 23.95,10.65 v24,10.2 | U100.R10 25.9,10.7 v25.8,10.2 | C107.1 19.2,21.4 v18.97,21.74 | 18.73,14.32 v18.42,14 | 28.93,13.68 29.6,13 v31,13 | U100.B5 17.32,14.32 16.8,13.8 15.5,13.8 | 27.69,13.8 28.2,13.8 28.4,14 | 28.6,14.32 27.52,14.32 | C112.1 19.8,31.2 | 28.8,32.4 28.73,32.4 | 14,18 13.88,18 13.88,17.93
  Bottom 0.3: 18.98,31.3 v18.36,31.31 | 19.48,29.39 v18.83,30.03 18.83,30.23 19.8,31.2 | 14,18 14.8,18 16.2,16.6 | v14.6,17.2 14.1,17.7 13.8,17.73 C106.1 | v22.25,27.37 21.2,27.37 C109.1 21.2,27 | v22.17,26.71 22.17,26.8 21.4,26.8 | C111.1 28.13,28.52 v28.13,27.58 | v28.13,26.86 28.1,26.86 28.1,27.6 | v27,27.4 26,27.4 C108.1
  Bottom 0.4: v29.2,30.61 29.2,31.4 28.6,32
  pour POW (isolate 0.17): 12,9.6 31,9.6 36.6,15.2 36.6,18.4 49.2,18.4 49.2,20.4 36.6,20.4 36.6,45.8 44.2,45.8 44.2,48.2 39.2,48.2 39.2,51 41.4,51 41.4,74.6 38.8,74.6 38.8,53 27.4,53 27.4,32 18.8,32 17.2,33.6 15.6,33.6 11.6,29.6 11.6,26.2 11.2,25.8 11.2,10.4
1.8V  (via drill 0.3, 0.4)
  Top 0.3: U8.5 43.92,17.77 | v17.1,17.5 17.1,18.18 C68.1
  Top 0.4: 43.92,17.77 C63.1 39.6,19.4 39,18.8 v39,12.4
  POW 0.2: v17.09,17.51 17.2,17.51 17.2,17.5 v17.1,17.5
  POW 0.8: 22.1,7.6 23.3,8.8
  POW 1: v17.09,17.51 17.09,16.49 15.6,15 15,15 14.2,14.2 14.2,11.78 v14.68,11.3 14.68,10.53 16.2,9 | 16.2,9 16.18,9 | 16.2,9 18.8,9 20.2,7.6 22.1,7.6 | 23.3,8.8 v25.84,8.8 v28.05,11.01 29.4,12.36 29.4,15.58 v30.62,16.8
  Bottom 0.11: 14.95,12.07 C102.1 14.8,12.2 | U100.R1 25.95,16.93 26.32,17.3 27.43,17.3 27.6,17.2 | C105.1 30.49,16.8 | 28.93,12.48 28.84,12.29 | C100.1 14.7,10.6 | 27.8,12.8 28,12.8 | 28.73,12 28.84,12.29 | C101.1 28.93,11.69 | 28.93,11.69 28.84,11.6 | 28.84,12.29 28.84,11.6 | 28.84,11.6 29.02,11.98 | 28.93,11.69 29.32,11.47
  Bottom 0.2: U100.C1 18.1,17.3 18,17.4 17.84,17.51 v17.1,17.5 | 27.6,17.2 28,16.8 | U100.B6 17.27,13.68 15.8,12.2 | 14.4,10.2 14.6,10.53 C100.1 | U100.T6 26.93,13.68 27.8,12.8
  Bottom 0.4: 28,16.8 C105.1 | 30.49,16.8 v30.62,16.8 | 28,12.8 28.4,12.4 28.73,12 | C102.1 v14.68,11.3 C100.1 | 29.02,11.98 v28.05,11.01 | 14.8,12.2 15.8,12.2 | 14.7,10.6 14.7,10.4
  Bottom 1: v25.84,8.8 28.05,8.8 | 28.05,8.8 31.6,8.8 35.2,12.4 v39,12.4 v39,13.6 | v28.05,11.01 28.05,8.8
3.3V  (via drill 0.3, 0.4)
  Top 0.2: U1.86 17.99,35.6 16,35.6 15.6,35 | 16.4,37.2 16.6,37.4 | C53.1 16.6,37.4 | 16.6,37.4 v17.2,37.4 17.6,37 18.29,37 U1.83 | 15.6,35 C56.1 15.4,35 | 15.6,35 v16.2,35 | 31,43 30.4,42.4 30.4,40.28 U1.56 | 31,43 31.12,43.12 | 31,43 v31,42.4 | v20.2,42.4 20.2,39.61 U1.75 | 20.25,45.27 R31.2 | U4.10 9.78,39.75 C51.1 | U6.8 U6.7 | RP1.1 v57,68.8 | R7.2 R8.2 R9.2 | R9.2 47.6,70.4 47.8,70.2 47.8,70.25 R9.2 | PWR.A 57,1.4 56,2.4 56,4 57,5 57,10 v55.2,11.8 | 55.45,19.32 C65.1
  Top 0.3: FB5.1 v45.4,48.6 | FB4.1 40.2,51 v40.2,50.1 | R7.2 v44,71.4 | R33.2 37.45,32.35 37.6,32.3 v37.6,31.5 | R34.2 49.35,37.75 49.1,37.8 v48.5,37.8 | C51.1 10.2,39.33 v10.2,38.4 | R37.2 v7,34.8 | C45.1 20.25,45.27 | C59.1 v39.8,27.8 | R56.2 36.85,10.15 v36.6,10.4 | 55.4,19.4 C65.1 55.52,20.07 v54.6,21 | 55.4,19.4 v54.6,19.4 | 55.4,19.4 v54.6,20.2 | 31.12,43.12 C49.1 | R58.2 44.65,10.15 44.4,10.4 v39,10.4 | R31.2 20.2,43.4 v20.2,42.4 v19.4,42.4
  Top 0.4: R46.2 v49.6,24 | R53.2 v6.8,12.8 | U10.5 55.45,19.32 | R62.2 v29.05,58.4 | R66.2 42.4,33.6 v41.5,33.6 | RP6.2 RP6.4 RP6.6 | RP6.8 RP6.6 | RP6.6 v53.2,29.6 | 44.4,23.2 U6.3 v44.44,21.4 | U6.8 41.9,27.5 41.27,26.88 C59.1
  Top 0.406: R54.2 v7.7,9.6
  Bottom 0.2: v55.2,11.8 55.2,18.6 v54.6,19.4
  Bottom 0.4: v31,42.4 v19.4,42.4 | 51.25,23.2 Q1.2 v51.25,22.4 | U11.5 50.55,36.58 C31.1 v49.6,36.6
  pour POW (isolate 0.4, rank 2): 60,85.6 0,85.6 0,61.2 8.2,61.2 8.2,59 4.8,59 4.8,46.8 10.4,46.8 10.4,44.8 5,44.8 5,7 7.6,4.2 40.4,4.2 40.2,16 55.2,16 55.2,45.4 60,45.4
+5V  (via drill 0.4)
  Top 0.2: C62.1 6.47,20.6 6.8,20.6 6.8,20.8
  Top 0.3: U10.3 57.35,13.95 57,13.6 55.6,13.6 55.4,13.8 55.4,15.05 U10.1 53.6,15.1 | 53.8,14.9 C71.1 53.62,15.12 53.6,15.1 | U9.3 51.55,13.75 51.2,13.4 49.8,13.4 49.6,13.6 49.6,15.05 | 49.6,15.05 U9.1 | 49.6,15.05 48.48,15.05 C72.1 48,15 v47.1,15 | v41.3,15.1 42,15.1 42,15.32 C70.1 42.62,15.1 U8.1 43.8,15.05 43.8,14 44.2,13.6 45.4,13.6 45.75,13.95 U8.3 | C46.1 10.47,45.8 | 10.47,45.8 v9.5,45.8 | v7.2,60.2 7.2,59.48 C26.1 7.8,59.27 7.8,60.6 6.97,61.42 U5.8 | U3.5 11.65,45.55 11.4,45.8 10.47,45.8 | 53.6,15.1 v52.9,15.1 | X1.1 v50.6,5.8 v50.6,5
  Top 0.4: U7.8 6.4,20.6 | 6.4,20.6 6.47,20.6 | 6.4,20.6 C62.1 6.4,18.6 4.2,16.4 UART_RV.P$1
  pour POW (isolate 0.4, rank 3): 0,61.2 60,61.2 60,0 0,0
BIAS1
  Top 0.2: U5.3 8.68,62.73 8.4,63 8.4,65.08 8.46,65.14 | 8.46,65.14 C18.1 8.55,65.22 R13.2 | U5.5 6.38,63.38 6.8,63.8 R15.2 8.45,65.15 8.46,65.14
CA0  (via drill 0.2)
  Top 0.11: v34,28 34,28.2 33.8,28.4 32.8,28.4 32.4,28.8 31.99,28.8 arc-45 31.29,29.09 30.91,29.09 29.77,30.23 29.78,30.61 29.78,30.78 29.4,31.11 29.27,31.11 U1.37
  Bottom 0.11: U100.P3 25.28,15.66 arc-45 25.99,15.95 31.62,15.95 arc90 34,18.32 34,18.85 arc-90 34.09,18.94 34.11,18.94 arc90 34.2,19.03 34.2,19.06 arc90 34.11,19.15 33.89,19.15 arc-90 33.8,19.25 33.8,19.27 arc-90 33.89,19.37 34.11,19.37 arc90 34.2,19.46 34.2,19.49 arc90 34.11,19.58 33.89,19.58 arc-90 33.8,19.67 33.8,19.7 arc-90 33.89,19.79 34.11,19.79 arc90 34.2,19.88 34.2,19.91 arc90 34.11,20 33.89,20 arc-90 33.8,20.1 33.8,20.13 arc-90 33.89,20.22 34.11,20.22 arc90 34.2,20.31 34.2,20.34 arc90 34.11,20.43 33.89,20.43 arc-90 33.8,20.52 33.8,20.55 arc-90 33.89,20.64 34.11,20.64 arc90 34.2,20.74 34.2,20.77 arc90 34.11,20.86 33.89,20.86 arc-90 33.8,20.95 33.8,20.98 arc-90 33.89,21.07 34.11,21.07 arc90 34.2,21.16 34.2,21.19 arc90 34.11,21.28 33.89,21.28 arc-90 33.8,21.37 33.8,21.4 arc-90 33.89,21.5 34.11,21.5 arc90 34.2,21.59 34.2,21.62 arc90 34.11,21.71 34.09,21.71 arc-90 34,21.8 v34,28
CA1  (via drill 0.2)
  Top 0.11: v34.8,26.8 34.8,27 34.6,27.2 33.6,27.2 33.2,27.6 32.06,27.6 arc-45 31.36,27.89 31.36,28.04 29.6,29.8 29.26,29.8 28.71,30.35 28.71,30.54 U1.35
  Bottom 0.11: U100.N3 24.63,15.59 arc45 25.34,15.3 31.62,15.3 arc90 34.8,18.48 34.8,20.2 arc-90 34.89,20.29 34.91,20.29 arc90 35,20.38 35,20.61 arc90 34.91,20.7 34.69,20.7 arc-90 34.6,20.79 34.6,21.02 arc-90 34.69,21.11 34.91,21.11 arc90 35,21.2 35,21.43 arc90 34.91,21.52 34.69,21.52 arc-90 34.6,21.61 34.6,21.84 arc-90 34.69,21.93 34.91,21.93 arc90 35,22.02 35,22.25 arc90 34.91,22.34 34.69,22.34 arc-90 34.6,22.43 34.6,22.66 arc-90 34.69,22.75 34.91,22.75 arc90 35,22.84 35,23.07 arc90 34.91,23.16 34.89,23.16 arc-90 34.8,23.25 v34.8,26.8
CA2  (via drill 0.2)
  Top 0.11: U1.34 31.74,26.94 31.88,26.8 33,26.8 33.8,26 35.4,26 35.6,25.8 v35.6,25.6
  Bottom 0.11: U100.M3 24.31,15.27 arc45 24.93,15.05 32.09,15.05 arc90 35.6,18.4 v35.6,25.6
CA3  (via drill 0.2)
  Top 0.11: U1.38 30.03,30.94 30.03,30.39 30.8,29.6 31.76,29.6 31.96,29.4 33,29.4 33.2,29.2 v33.2,29
  Bottom 0.11: U100.M2 23.98,16.31 arc45 24.27,17.01 24.27,17.07 arc-90 24.8,17.6 31.2,17.6 arc90 33.2,19.6 33.2,19.8 arc-90 33.29,19.89 33.32,19.89 arc90 33.41,19.99 33.41,19.99 arc90 33.32,20.08 33.08,20.08 arc-90 32.98,20.17 32.98,20.17 arc-90 33.08,20.27 33.32,20.27 arc90 33.41,20.36 33.41,20.36 arc90 33.32,20.45 33.08,20.45 arc-90 32.98,20.54 32.98,20.55 arc-90 33.08,20.64 33.32,20.64 arc90 33.41,20.73 33.41,20.73 arc90 33.32,20.82 33.08,20.82 arc-90 32.98,20.91 32.98,20.92 arc-90 33.08,21.01 33.32,21.01 arc90 33.41,21.1 33.41,21.1 arc90 33.32,21.19 33.08,21.19 arc-90 32.98,21.29 32.98,21.29 arc-90 33.08,21.38 33.32,21.38 arc90 33.41,21.47 33.41,21.47 arc90 33.32,21.57 33.08,21.57 arc-90 32.98,21.66 32.98,21.66 arc-90 33.08,21.75 33.32,21.75 arc90 33.41,21.84 33.41,21.84 arc90 33.32,21.94 33.08,21.94 arc-90 32.98,22.03 32.98,22.03 arc-90 33.08,22.12 33.32,22.12 arc90 33.41,22.21 33.41,22.22 arc90 33.32,22.31 33.29,22.31 arc-90 33.2,22.4 v33.2,29
CA4  (via drill 0.2)
  Top 0.11: v32.4,30 32.2,30.2 32.12,30.2 31.87,29.93 30.87,29.93 30.29,30.53 30.29,30.73 30.29,31.24 U1.39
  Bottom 0.11: U100.M1 23.95,17.15 arc-90 24.8,18 30.8,18 arc90 32.4,19.6 32.4,19.96 arc-90 32.49,20.05 32.55,20.05 arc90 32.64,20.14 32.64,20.15 arc90 32.55,20.24 32.25,20.24 arc-90 32.16,20.33 32.16,20.34 arc-90 32.25,20.43 32.55,20.43 arc90 32.64,20.52 32.64,20.53 arc90 32.55,20.62 32.25,20.62 arc-90 32.16,20.71 32.16,20.72 arc-90 32.25,20.81 32.55,20.81 arc90 32.64,20.9 32.64,20.91 arc90 32.55,21 32.25,21 arc-90 32.16,21.09 32.16,21.1 arc-90 32.25,21.19 32.55,21.19 arc90 32.64,21.29 32.64,21.29 arc90 32.55,21.38 32.25,21.38 arc-90 32.16,21.48 32.16,21.48 arc-90 32.25,21.57 32.55,21.57 arc90 32.64,21.67 32.64,21.67 arc90 32.55,21.76 32.25,21.76 arc-90 32.16,21.86 32.16,21.86 arc-90 32.25,21.95 32.55,21.95 arc90 32.64,22.05 32.64,22.05 arc90 32.55,22.15 32.25,22.15 arc-90 32.16,22.24 32.16,22.24 arc-90 32.25,22.34 32.55,22.34 arc90 32.64,22.43 32.64,22.43 arc90 32.55,22.53 32.25,22.53 arc-90 32.16,22.62 32.16,22.62 arc-90 32.25,22.72 32.55,22.72 arc90 32.64,22.81 32.64,22.82 arc90 32.55,22.91 32.49,22.91 arc-90 32.4,23 v32.4,30
CA5  (via drill 0.2)
  Top 0.11: v16.6,33 16.8,33.2 17.6,33.2 17.83,33.43 U1.1
  Bottom 0.11: U100.G2 20.67,16.31 arc-45 20.38,17.01 20.38,18.02 arc90 18.8,19.6 17.2,19.6 arc-90 16.4,20.4 16.4,21.53 arc-90 16.49,21.62 16.75,21.62 arc90 16.84,21.71 16.84,21.72 arc90 16.75,21.82 16.49,21.82 arc-90 16.4,21.91 16.4,21.92 arc-90 16.49,22.01 16.75,22.01 arc90 16.84,22.1 16.84,22.11 arc90 16.75,22.21 16.49,22.21 arc-90 16.4,22.3 16.4,22.31 arc-90 16.49,22.4 16.75,22.4 arc90 16.84,22.5 16.84,22.51 arc90 16.75,22.6 16.49,22.6 arc-90 16.4,22.69 16.4,22.7 arc-90 16.49,22.79 16.75,22.79 arc90 16.84,22.89 16.84,22.9 arc90 16.75,22.99 16.49,22.99 arc-90 16.4,23.08 16.4,23.09 arc-90 16.49,23.18 16.75,23.18 arc90 16.84,23.28 16.84,23.29 arc90 16.75,23.38 16.49,23.38 arc-90 16.4,23.47 16.4,23.48 arc-90 16.49,23.58 16.75,23.58 arc90 16.84,23.67 16.84,23.68 arc90 16.75,23.77 16.49,23.77 arc-90 16.4,23.86 16.4,23.88 arc-90 16.49,23.97 16.75,23.97 arc90 16.84,24.06 16.84,24.07 arc90 16.75,24.16 16.49,24.16 arc-90 16.4,24.25 16.4,24.27 arc-90 16.49,24.36 16.75,24.36 arc90 16.84,24.45 16.84,24.46 arc90 16.75,24.55 16.49,24.55 arc-90 16.4,24.64 16.4,24.66 arc-90 16.49,24.75 16.75,24.75 arc90 16.84,24.84 16.84,24.85 arc90 16.75,24.94 16.49,24.94 arc-90 16.4,25.04 16.4,25.05 arc-90 16.49,25.14 16.75,25.14 arc90 16.84,25.23 16.84,25.24 arc90 16.75,25.34 16.49,25.34 arc-90 16.4,25.43 16.4,25.44 arc-90 16.49,25.53 16.75,25.53 arc90 16.84,25.62 16.84,25.63 arc90 16.75,25.73 16.49,25.73 arc-90 16.4,25.82 16.4,25.83 arc-90 16.49,25.92 16.75,25.92 arc90 16.84,26.01 16.84,26.02 arc90 16.75,26.12 16.49,26.12 arc-90 16.4,26.21 16.4,26.22 arc-90 16.49,26.31 16.75,26.31 arc90 16.84,26.41 16.84,26.42 arc90 16.75,26.51 16.49,26.51 arc-90 16.4,26.6 16.4,32.8 v16.6,33
CA6  (via drill 0.2)
  Top 0.11: v15.6,32 15.6,32.2 15.8,32.4 16.8,32.4 16.95,32.4 17.22,32.67 17.7,32.67 U1.2
  Bottom 0.11: U100.F2 20.02,16.31 20.02,16.46 19.74,16.74 19.74,17.12 19.8,17.18 19.8,17.68 19.28,18.2 18.68,18.8 18.4,18.8 16.8,18.8 arc-90 15.6,20 15.6,21.53 arc-90 15.69,21.62 15.9,21.62 arc90 15.99,21.71 15.99,21.72 arc90 15.9,21.81 15.69,21.81 arc-90 15.6,21.9 15.6,21.91 arc-90 15.69,22 15.9,22 arc90 15.99,22.09 15.99,22.09 arc90 15.9,22.19 15.69,22.19 arc-90 15.6,22.28 15.6,22.28 arc-90 15.69,22.38 15.9,22.38 arc90 15.99,22.47 15.99,22.47 arc90 15.9,22.56 15.69,22.56 arc-90 15.6,22.66 15.6,22.66 arc-90 15.69,22.75 15.9,22.75 arc90 15.99,22.84 15.99,22.85 arc90 15.9,22.94 15.69,22.94 arc-90 15.6,23.03 15.6,23.04 arc-90 15.69,23.13 15.9,23.13 arc90 15.99,23.22 15.99,23.23 arc90 15.9,23.32 15.69,23.32 arc-90 15.6,23.41 15.6,23.41 arc-90 15.69,23.5 15.9,23.5 arc90 15.99,23.6 15.99,23.6 arc90 15.9,23.69 15.69,23.69 arc-90 15.6,23.79 15.6,23.79 arc-90 15.69,23.88 15.9,23.88 arc90 15.99,23.97 15.99,23.98 arc90 15.9,24.07 15.69,24.07 arc-90 15.6,24.16 15.6,24.17 arc-90 15.69,24.26 15.9,24.26 arc90 15.99,24.35 15.99,24.36 arc90 15.9,24.45 15.69,24.45 arc-90 15.6,24.54 15.6,24.54 arc-90 15.69,24.64 15.9,24.64 arc90 15.99,24.73 15.99,24.73 arc90 15.9,24.82 15.69,24.82 arc-90 15.6,24.92 15.6,24.92 arc-90 15.69,25.01 15.9,25.01 arc90 15.99,25.1 15.99,25.11 arc90 15.9,25.2 15.69,25.2 arc-90 15.6,25.29 15.6,25.3 arc-90 15.69,25.39 15.9,25.39 arc90 15.99,25.48 15.99,25.49 arc90 15.9,25.58 15.69,25.58 arc-90 15.6,25.67 15.6,25.67 arc-90 15.69,25.77 15.9,25.77 arc90 15.99,25.86 15.99,25.86 arc90 15.9,25.95 15.69,25.95 arc-90 15.6,26.05 15.6,26.05 arc-90 15.69,26.14 15.9,26.14 arc90 15.99,26.23 15.99,26.24 arc90 15.9,26.33 15.69,26.33 arc-90 15.6,26.42 15.6,26.43 arc-90 15.69,26.52 15.9,26.52 arc90 15.99,26.61 15.99,26.62 arc90 15.9,26.71 15.69,26.71 arc-90 15.6,26.8 v15.6,32
CA7  (via drill 0.2)
  Top 0.11: v12.4,29.6 arc-45 13.37,30 14.76,30 arc45 16.53,30.73 17.6,31.8 18.52,31.8 U1.5
  Bottom 0.11: U100.F3 19.48,15.05 15.38,15.05 arc-90 12.4,18 12.4,21.76 arc90 12.22,21.94 12.19,21.94 arc-90 12.01,22.12 12.01,22.17 arc-90 12.19,22.35 12.22,22.35 arc90 12.4,22.53 12.4,22.59 arc90 12.22,22.77 12.19,22.77 arc-90 12.01,22.95 12.01,23 arc-90 12.19,23.18 12.22,23.18 arc90 12.4,23.36 12.4,23.41 arc90 12.22,23.59 12.19,23.59 arc-90 12.01,23.77 12.01,23.82 arc-90 12.19,24 12.22,24 arc90 12.4,24.18 12.4,24.23 arc90 12.22,24.41 12.19,24.41 arc-90 12.01,24.59 12.01,24.64 arc-90 12.19,24.82 12.22,24.82 arc90 12.4,25 v12.4,29.6
CA8  (via drill 0.2)
  Top 0.11: v13.2,30.4 arc-45 14.17,30.8 15.16,30.8 arc45 16.93,31.53 17.46,32.06 18.22,32.06 U1.4
  Bottom 0.11: U100.E3 19.37,15.59 arc-45 18.66,15.3 15.7,15.3 arc-90 12.8,18.4 12.8,20.8 arc-45 12.94,21.14 13.06,21.26 arc45 13.2,21.6 13.2,21.8 arc-90 13.38,21.98 13.55,21.98 arc90 13.73,22.16 13.73,22.23 arc90 13.55,22.41 13.38,22.41 arc-90 13.2,22.59 13.2,22.67 arc-90 13.38,22.85 13.55,22.85 arc90 13.73,23.03 13.73,23.1 arc90 13.55,23.28 13.38,23.28 arc-90 13.2,23.46 13.2,23.53 arc-90 13.38,23.71 13.55,23.71 arc90 13.73,23.89 13.73,23.96 arc90 13.55,24.14 13.38,24.14 arc-90 13.2,24.32 13.2,24.4 arc-90 13.38,24.58 13.55,24.58 arc90 13.73,24.76 13.73,24.83 arc90 13.55,25.01 13.38,25.01 arc-90 13.2,25.19 13.2,25.26 arc-90 13.38,25.44 13.55,25.44 arc90 13.73,25.62 13.73,25.7 arc90 13.55,25.88 13.38,25.88 arc-90 13.2,26.05 v13.2,30.4
CA9  (via drill 0.2)
  Top 0.11: v14.8,31.2 14.8,31.4 15,31.6 16.6,31.6 17.4,32.4 17.99,32.4 U1.3
  Bottom 0.11: U100.E2 19.37,16.31 19.37,16.44 19.08,16.73 19.08,17.09 18.9,17.25 18.9,17.5 18.4,18 16,18 arc-90 14.8,19.2 14.8,21.25 arc-90 14.89,21.34 14.9,21.34 arc90 15,21.43 15,21.45 arc90 14.9,21.54 14.7,21.54 arc-90 14.6,21.63 14.6,21.65 arc-90 14.7,21.74 14.9,21.74 arc90 15,21.83 15,21.85 arc90 14.9,21.94 14.7,21.94 arc-90 14.6,22.03 14.6,22.04 arc-90 14.7,22.14 14.9,22.14 arc90 15,22.23 15,22.24 arc90 14.9,22.34 14.7,22.34 arc-90 14.6,22.43 14.6,22.44 arc-90 14.7,22.53 14.9,22.53 arc90 15,22.63 15,22.64 arc90 14.9,22.73 14.7,22.73 arc-90 14.6,22.82 14.6,22.84 arc-90 14.7,22.93 14.9,22.93 arc90 15,23.02 15,23.04 arc90 14.9,23.13 14.7,23.13 arc-90 14.6,23.22 14.6,23.24 arc-90 14.7,23.33 14.9,23.33 arc90 15,23.42 15,23.43 arc90 14.9,23.53 14.7,23.53 arc-90 14.6,23.62 14.6,23.63 arc-90 14.7,23.73 14.9,23.73 arc90 15,23.82 15,23.83 arc90 14.9,23.92 14.7,23.92 arc-90 14.6,24.02 14.6,24.03 arc-90 14.7,24.12 14.9,24.12 arc90 15,24.21 15,24.23 arc90 14.9,24.32 14.7,24.32 arc-90 14.6,24.41 14.6,24.43 arc-90 14.7,24.52 14.9,24.52 arc90 15,24.61 15,24.63 arc90 14.9,24.72 14.7,24.72 arc-90 14.6,24.81 14.6,24.82 arc-90 14.7,24.92 14.9,24.92 arc90 15,25.01 15,25.02 arc90 14.9,25.12 14.7,25.12 arc-90 14.6,25.21 14.6,25.22 arc-90 14.7,25.32 14.9,25.32 arc90 15,25.41 15,25.42 arc90 14.9,25.51 14.7,25.51 arc-90 14.6,25.61 14.6,25.62 arc-90 14.7,25.71 14.9,25.71 arc90 15,25.8 15,25.82 arc90 14.9,25.91 14.7,25.91 arc-90 14.6,26 14.6,26.02 arc-90 14.7,26.11 14.9,26.11 arc90 15,26.2 15,26.22 arc90 14.9,26.31 14.89,26.31 arc-90 14.8,26.4 v14.8,31.2
CKB  (via drill 0.2)
  Top 0.11: U1.41 30.51,32.14 31.2,31.44 v31.2,31
  Bottom 0.11: U100.J3 22.03,15.66 arc45 22.32,16.36 22.32,17.57 22.32,19.52 23.3,20.5 | v31.2,31 arc-90 30.6,30.4 arc90 30.2,30 30.2,29 arc90 30.3,28.9 30.37,28.9 arc-90 30.47,28.8 30.47,28.78 arc-90 30.37,28.68 30.03,28.68 arc90 29.93,28.58 29.93,28.56 arc90 30.03,28.46 30.37,28.46 arc-90 30.47,28.36 30.47,28.34 arc-90 30.37,28.24 30.03,28.24 arc90 29.93,28.14 29.93,28.12 arc90 30.03,28.02 30.37,28.02 arc-90 30.47,27.92 30.47,27.9 arc-90 30.37,27.8 30.03,27.8 arc90 29.93,27.7 29.93,27.68 arc90 30.03,27.58 30.37,27.58 arc-90 30.47,27.48 30.47,27.46 arc-90 30.37,27.36 30.03,27.36 arc90 29.93,27.26 29.93,27.24 arc90 30.03,27.14 30.37,27.14 arc-90 30.47,27.04 30.47,27.02 arc-90 30.37,26.92 30.03,26.92 arc90 29.93,26.82 29.93,26.8 arc90 30.03,26.7 30.37,26.7 arc-90 30.47,26.6 30.47,26.58 arc-90 30.37,26.48 30.03,26.48 arc90 29.93,26.38 29.93,26.36 arc90 30.03,26.26 30.37,26.26 arc-90 30.47,26.16 30.47,26.14 arc-90 30.37,26.04 30.03,26.04 arc90 29.93,25.93 29.93,25.91 arc90 30.03,25.82 30.37,25.82 arc-90 30.47,25.71 30.47,25.7 arc-90 30.37,25.59 30.3,25.59 arc90 30.2,25.5 30.2,23.8 30.2,21.8 29.8,21.4 29.2,20.8 28.67,20.8 27.4,20.8 24.46,20.8 24.23,20.8 23.6,20.8 23.3,20.5 | R100.1 23.25,20.55 23.3,20.5
CKEB  (via drill 0.2)
  Top 0.11: U1.33 30.8,27.32 31.2,26.92 31.2,26 31.2,25.8 | 31.2,25.8 31.2,25.4 31,25.2 v30.8,25.2 | R45.2 31.25,25.85 31.2,25.8
  Bottom 0.11: U100.K1 22.65,17.05 arc-90 24.4,18.8 29,18.8 29.2,18.8 30.2,19.8 30.51,19.8 30.8,20.09 arc-90 30.9,20.19 30.96,20.19 arc90 31.06,20.29 31.06,20.31 arc90 30.96,20.41 30.64,20.41 arc-90 30.54,20.51 30.54,20.52 arc-90 30.64,20.62 30.96,20.62 arc90 31.06,20.72 31.06,20.73 arc90 30.96,20.84 30.64,20.84 arc-90 30.54,20.93 30.54,20.95 arc-90 30.64,21.05 30.96,21.05 arc90 31.06,21.15 31.06,21.16 arc90 30.96,21.27 30.64,21.27 arc-90 30.54,21.36 30.54,21.38 arc-90 30.64,21.48 30.96,21.48 arc90 31.06,21.58 31.06,21.59 arc90 30.96,21.69 30.64,21.69 arc-90 30.54,21.79 30.54,21.81 arc-90 30.64,21.91 30.96,21.91 arc90 31.06,22.01 31.06,22.02 arc90 30.96,22.12 30.64,22.12 arc-90 30.54,22.22 30.54,22.24 arc-90 30.64,22.34 30.96,22.34 arc90 31.06,22.44 31.06,22.45 arc90 30.96,22.55 30.64,22.55 arc-90 30.54,22.65 30.54,22.67 arc-90 30.64,22.77 30.96,22.77 arc90 31.06,22.87 31.06,22.88 arc90 30.96,22.98 30.64,22.98 arc-90 30.54,23.08 30.54,23.1 arc-90 30.64,23.2 30.96,23.2 arc90 31.06,23.3 31.06,23.31 arc90 30.96,23.41 30.64,23.41 arc-90 30.54,23.51 30.54,23.53 arc-90 30.64,23.63 30.96,23.63 arc90 31.06,23.73 31.06,23.74 arc90 30.96,23.84 30.64,23.84 arc-90 30.54,23.94 30.54,23.96 arc-90 30.64,24.06 30.96,24.06 arc90 31.06,24.16 31.06,24.17 arc90 30.96,24.27 30.64,24.27 arc-90 30.54,24.37 30.54,24.39 arc-90 30.64,24.48 30.96,24.48 arc90 31.06,24.59 31.06,24.6 arc90 30.96,24.7 30.9,24.7 arc-90 30.8,24.8 v30.8,25.2
CSXB  (via drill 0.2)
  Top 0.11: v31.6,30.4 arc45 30.73,30.57 30.6,30.7 30.6,31.48 30.11,31.97 U1.40
  Bottom 0.11: U100.L1 23.3,17.3 arc-90 24.4,18.4 30.4,18.4 arc90 31.6,19.6 31.6,22.4 arc-90 31.7,22.5 31.71,22.5 arc90 31.81,22.6 31.81,22.72 arc90 31.71,22.82 31.49,22.82 arc-90 31.39,22.92 31.39,23.04 arc-90 31.49,23.14 31.71,23.14 arc90 31.81,23.24 31.81,23.36 arc90 31.71,23.46 31.49,23.46 arc-90 31.39,23.56 31.39,23.68 arc-90 31.49,23.78 31.71,23.78 arc90 31.81,23.88 31.81,24 arc90 31.71,24.1 31.49,24.1 arc-90 31.39,24.2 31.39,24.32 arc-90 31.49,24.42 31.71,24.42 arc90 31.81,24.52 31.81,24.64 arc90 31.71,24.74 31.49,24.74 arc-90 31.39,24.84 31.39,24.96 arc-90 31.49,25.06 31.71,25.06 arc90 31.81,25.16 31.81,25.28 arc90 31.71,25.38 31.49,25.38 arc-90 31.39,25.48 31.39,25.6 arc-90 31.49,25.7 31.71,25.7 arc90 31.81,25.8 31.81,25.92 arc90 31.71,26.02 31.49,26.02 arc-90 31.39,26.12 31.39,26.24 arc-90 31.49,26.34 31.71,26.34 arc90 31.81,26.44 31.81,26.55 arc90 31.71,26.66 31.49,26.66 arc-90 31.39,26.75 31.39,26.88 arc-90 31.49,26.98 31.71,26.98 arc90 31.81,27.07 31.81,27.2 arc90 31.71,27.3 31.49,27.3 arc-90 31.39,27.39 31.39,27.51 arc-90 31.49,27.61 31.71,27.61 arc90 31.81,27.71 31.81,27.83 arc90 31.71,27.93 31.49,27.93 arc-90 31.39,28.03 31.39,28.15 arc-90 31.49,28.25 31.71,28.25 arc90 31.81,28.35 31.81,28.47 arc90 31.71,28.57 31.49,28.57 arc-90 31.39,28.67 31.39,28.79 arc-90 31.49,28.89 31.71,28.89 arc90 31.81,28.99 31.81,29.11 arc90 31.71,29.21 31.7,29.21 arc-90 31.6,29.31 v31.6,30.4
D0  (via drill 0.2)
  Top 0.11: 29.79,15.19 arc90 29.89,15.09 30.11,15.09 arc-90 30.21,14.99 30.21,14.99 arc-90 30.11,14.89 30.1,14.89 arc90 30,14.79 30,14.45 arc-90 26.95,11.4 v24.93,11.4 | 29.79,15.19 | 29.79,15.19 arc-90 29.89,15.29 30.11,15.29 arc90 30.21,15.39 30.21,15.39 arc90 30.11,15.49 29.89,15.49 arc-90 29.79,15.59 | 29.79,15.59 | 29.79,15.59 arc-90 29.89,15.69 30.11,15.69 arc90 30.21,15.79 30.21,15.79 arc90 30.11,15.89 29.89,15.89 arc-90 29.79,15.99 | 29.79,15.99 | 29.79,15.99 arc-90 29.89,16.09 30.11,16.09 arc90 30.21,16.19 30.21,16.19 arc90 30.11,16.29 29.89,16.29 arc-90 29.79,16.39 | 29.79,16.39 | 29.79,16.39 arc-90 29.89,16.49 30.11,16.49 arc90 30.21,16.59 30.21,16.59 arc90 30.11,16.7 29.89,16.7 arc-90 29.79,16.8 | 29.79,16.8 | 29.79,16.8 arc-90 29.89,16.89 30.11,16.89 arc90 30.21,17 30.21,17 arc90 30.11,17.1 29.89,17.1 arc-90 29.79,17.2 | 29.79,17.2 | 29.79,17.2 arc-90 29.89,17.3 30.11,17.3 arc90 30.21,17.4 30.21,17.4 arc90 30.11,17.5 29.89,17.5 arc-90 29.79,17.6 | 29.79,17.6 | 29.79,17.6 arc-90 29.89,17.7 30.11,17.7 arc90 30.21,17.8 30.21,17.8 arc90 30.11,17.9 29.89,17.9 arc-90 29.79,18 | 29.79,18 | 29.79,18 arc-90 29.89,18.1 30.11,18.1 arc90 30.21,18.2 30.21,18.2 arc90 30.11,18.3 29.89,18.3 arc-90 29.79,18.4 | 29.79,18.4 | 29.79,18.4 arc-90 29.89,18.5 30.11,18.5 arc90 30.21,18.6 30.21,18.6 arc90 30.11,18.7 30.1,18.7 arc-90 30,18.8 TP_D5.TP | U1.32 30,27.55 30,26.6 | TP_D5.TP 30,26.6 | TP_D5.TP 30,26.6
  Bottom 0.11: U100.N8 24.63,12.34 arc-45 24.93,11.64 v24.93,11.4
D1  (via drill 0.2)
  Top 0.11: v24.27,12.05 26.8,12.05 arc90 29.2,14.45 29.2,14.56 arc-90 29.3,14.66 29.3,14.66 arc90 29.4,14.76 29.4,14.76 arc90 29.3,14.86 29.1,14.86 arc-90 29,14.96 29,14.96 arc-90 29.1,15.06 29.3,15.06 arc90 29.4,15.16 29.4,15.16 arc90 29.3,15.26 29.1,15.26 arc-90 29,15.36 29,15.37 arc-90 29.1,15.46 29.3,15.46 arc90 29.4,15.56 29.4,15.57 arc90 29.3,15.67 29.1,15.67 arc-90 29,15.77 29,15.77 arc-90 29.1,15.87 29.3,15.87 arc90 29.4,15.97 29.4,15.97 arc90 29.3,16.07 29.1,16.07 arc-90 29,16.17 29,16.17 arc-90 29.1,16.27 29.3,16.27 arc90 29.4,16.37 29.4,16.37 arc90 29.3,16.47 29.1,16.47 arc-90 29,16.57 29,16.57 arc-90 29.1,16.68 29.3,16.68 arc90 29.4,16.77 29.4,16.78 arc90 29.3,16.88 29.1,16.88 arc-90 29,16.98 29,16.98 arc-90 29.1,17.08 29.3,17.08 arc90 29.4,17.18 29.4,17.18 arc90 29.3,17.28 29.1,17.28 arc-90 29,17.38 29,17.38 arc-90 29.1,17.48 29.3,17.48 arc90 29.4,17.58 29.4,17.58 arc90 29.3,17.68 29.1,17.68 arc-90 29,17.78 29,17.79 arc-90 29.1,17.89 29.3,17.89 arc90 29.4,17.98 29.4,17.99 arc90 29.3,18.09 29.1,18.09 arc-90 29,18.19 29,18.19 arc-90 29.1,18.29 29.3,18.29 arc90 29.4,18.39 29.4,18.39 arc90 29.3,18.49 29.1,18.49 arc-90 29,18.59 29,18.59 arc-90 29.1,18.69 29.3,18.69 arc90 29.4,18.79 29.4,18.79 arc90 29.3,18.89 29.1,18.89 arc-90 29,18.99 29,19 arc-90 29.1,19.09 29.3,19.09 arc90 29.4,19.2 29.4,19.2 arc90 29.3,19.3 29.1,19.3 arc-90 29,19.4 29,19.4 arc-90 29.1,19.5 29.3,19.5 arc90 29.4,19.6 29.4,19.6 arc90 29.3,19.7 29.3,19.7 arc-90 29.2,19.8 29.2,20.6 29.6,21 29.6,22 29.2,22.4 29.2,24.2
  Top 0.11: U1.31 29.2,27.79 29.2,26.4 29.2,25 29.2,24.2 | TP_D13.TP 29.24,24.24 29.2,24.2
  Bottom 0.11: U100.M8 v24.27,12.05
D2  (via drill 0.2)
  Top 0.11: v24.27,12.7 26.65,12.7 arc90 28.4,14.45 28.4,14.79 arc-90 28.5,14.89 28.5,14.89 arc90 28.6,14.99 28.6,15.07 arc90 28.5,15.17 28.3,15.17 arc-90 28.2,15.27 28.2,15.36 arc-90 28.3,15.46 28.5,15.46 arc90 28.6,15.56 28.6,15.64 arc90 28.5,15.74 28.3,15.74 arc-90 28.2,15.84 28.2,15.92 arc-90 28.3,16.02 28.5,16.02 arc90 28.6,16.12 28.6,16.21 arc90 28.5,16.31 28.3,16.31 arc-90 28.2,16.41 28.2,16.49 arc-90 28.3,16.59 28.5,16.59 arc90 28.6,16.69 28.6,16.77 arc90 28.5,16.87 28.3,16.87 arc-90 28.2,16.97 28.2,17.05 arc-90 28.3,17.16 28.5,17.16 arc90 28.6,17.25 28.6,17.34 arc90 28.5,17.44 28.3,17.44 arc-90 28.2,17.54 28.2,17.62 arc-90 28.3,17.72 28.5,17.72 arc90 28.6,17.82 28.6,17.9 arc90 28.5,18 28.3,18 arc-90 28.2,18.1 28.2,18.19 arc-90 28.3,18.29 28.5,18.29 arc90 28.6,18.39 28.6,18.47 arc90 28.5,18.57 28.3,18.57 arc-90 28.2,18.67 28.2,18.75 arc-90 28.3,18.85 28.5,18.85 arc90 28.6,18.95 28.6,19.04 arc90 28.5,19.14 28.3,19.14 arc-90 28.2,19.24 28.2,19.32 arc-90 28.3,19.42 28.5,19.42 arc90 28.6,19.52 28.6,19.6 arc90 28.5,19.7 28.3,19.7 arc-90 28.2,19.8 28.2,19.89 arc-90 28.3,19.99 28.5,19.99 arc90 28.6,20.09 28.6,20.17 arc90 28.5,20.27 28.3,20.27 arc-90 28.2,20.37 28.2,20.45 arc-90 28.3,20.55 28.5,20.55 arc90 28.6,20.65 28.6,20.73 arc90 28.5,20.84 28.3,20.84 arc-90 28.2,20.93 28.2,21.02 arc-90 28.3,21.12 28.5,21.12 arc90 28.6,21.22 28.6,21.3 arc90 28.5,21.4 28.3,21.4 arc-90 28.2,21.5 28.2,21.59 arc-90 28.3,21.68 28.5,21.68 arc90 28.6,21.79 28.6,21.87 arc90 28.5,21.97 28.3,21.97 arc-90 28.2,22.07 28.2,22.15 arc-90 28.3,22.25 28.5,22.25 arc90 28.6,22.35 28.6,22.43 arc90 28.5,22.53 28.3,22.53 arc-90 28.2,22.63 28.2,22.72 arc-90 28.3,22.82 28.5,22.82 arc90 28.6,22.92 28.6,23 arc90 28.5,23.1 28.5,23.1 arc-90 28.4,23.2 28.4,26
  Top 0.11: 28.4,26 28.4,26.2 28.6,26.4 28.6,28 28.4,28.2 28.2,28.2 26.95,29.45 U1.30 | TP_D9.TP 28.39,25.99 28.4,26
  Bottom 0.11: U100.M7 v24.27,12.7
D3  (via drill 0.2)
  Top 0.11: 27.6,24.8 27.6,24.2 arc90 27.7,24.1 27.71,24.1 arc-90 27.81,24 27.81,23.95 arc-90 27.71,23.85 27.49,23.85 arc90 27.39,23.75 27.39,23.7 arc90 27.49,23.6 27.71,23.6 arc-90 27.81,23.5 27.81,23.45 arc-90 27.71,23.35 27.49,23.35 arc90 27.39,23.25 27.39,23.2 arc90 27.49,23.1 27.71,23.1 arc-90 27.81,23 27.81,22.95 arc-90 27.71,22.85 27.49,22.85 arc90 27.39,22.75 27.39,22.7 arc90 27.49,22.61 27.71,22.61 arc-90 27.81,22.5 27.81,22.46 arc-90 27.71,22.36 27.49,22.36 arc90 27.39,22.26 27.39,22.21 arc90 27.49,22.11 27.71,22.11 arc-90 27.81,22.01 27.81,21.96 arc-90 27.71,21.86 27.49,21.86 arc90 27.39,21.76 27.39,21.71 arc90 27.49,21.61 27.71,21.61 arc-90 27.81,21.51 27.81,21.46 arc-90 27.71,21.36 27.49,21.36 arc90 27.39,21.26 27.39,21.21 arc90 27.49,21.11 27.71,21.11 arc-90 27.81,21.01 27.81,20.96 arc-90 27.71,20.86 27.49,20.86 arc90 27.39,20.76 27.39,20.71 arc90 27.49,20.61 27.71,20.61 arc-90 27.81,20.51 27.81,20.46 arc-90 27.71,20.36 27.49,20.36 arc90 27.39,20.26 27.39,20.21 arc90 27.49,20.11 27.71,20.11 arc-90 27.81,20.01 27.81,19.96 arc-90 27.71,19.86 27.49,19.86 arc90 27.39,19.76 27.39,19.71 arc90 27.49,19.61 27.71,19.61 arc-90 27.81,19.51 27.81,19.46 arc-90 27.71,19.36 27.49,19.36 arc90 27.39,19.27 27.39,19.22 arc90 27.49,19.12 27.71,19.12 arc-90 27.81,19.02 27.81,18.97 arc-90 27.71,18.87 27.49,18.87 arc90 27.39,18.77 27.39,18.72 arc90 27.49,18.62 27.71,18.62 arc-90 27.81,18.52 27.81,18.47 arc-90 27.71,18.37 27.49,18.37 arc90 27.39,18.27 27.39,18.22 arc90 27.49,18.12 27.71,18.12 arc-90 27.81,18.02 27.81,17.97 arc-90 27.71,17.87 27.49,17.87 arc90 27.39,17.77 27.39,17.72 arc90 27.49,17.62 27.71,17.62 arc-90 27.81,17.52 27.81,17.47 arc-90 27.71,17.37 27.49,17.37 arc90 27.39,17.27 27.39,17.22 arc90 27.49,17.12 27.71,17.12 arc-90 27.81,17.02 27.81,16.97 arc-90 27.71,16.87 27.49,16.87 arc90 27.39,16.77 27.39,16.72 arc90 27.49,16.62 27.71,16.62 arc-90 27.81,16.52 27.81,16.48 arc-90 27.71,16.38 27.7,16.38 arc90 27.6,16.27 27.6,15.25 arc-90 25.7,13.35 24.69,13.35 arc90 23.62,12.29 v23.62,12.05
  Top 0.11: 27.6,24.8 27.6,26.4 27.6,27.6 27.49,27.8 U1.28 | TP_D12.TP 27.61,24.81 27.6,24.8
  Bottom 0.11: U100.M9 v23.62,12.05
D4  (via drill 0.2)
